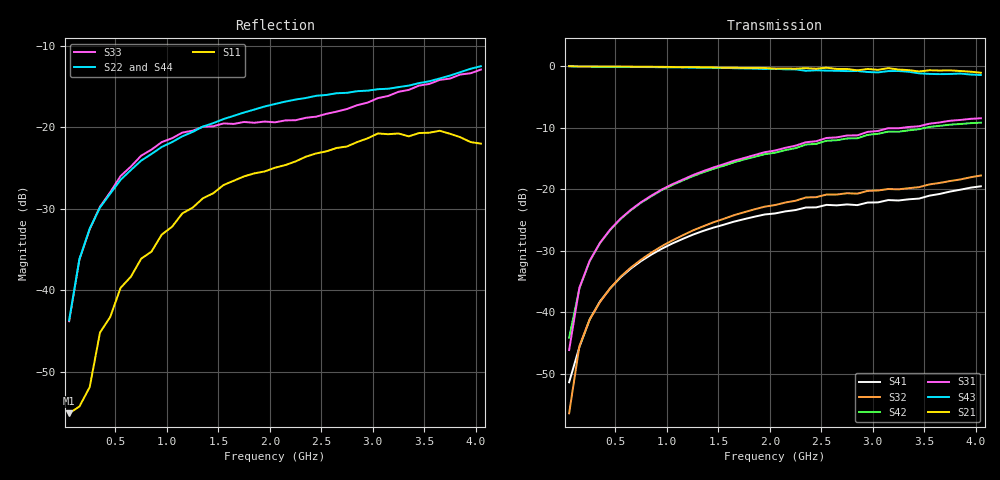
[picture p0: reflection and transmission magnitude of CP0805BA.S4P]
! Network Analyzer HP8720D.07.14 Serial No. US38111185
! 28 Apr 1999  02:06:29
! Frequency 	S11		S21		S31		S41		S12		S22		S23		S24		S13		S23		S33		S34		S14		S24		S34		S44
# HZ  S  DB R 50
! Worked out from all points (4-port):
!   41 points, 50 MHz to 4.05 GHz, reference 50 ohm
!   strongest paths, dB at 50 MHz, 1.05 GHz, 2.05 GHz, 3.05 GHz, 4.05 GHz:
!     S21: 0.0, -0.1, -0.4, -0.6, -1.0
!     S43: 0.0, -0.2, -0.4, -1.0, -1.4
!     S31: -46.1, -19.2, -13.7, -10.5, -8.4
!     S42: -44.1, -19.3, -14.0, -11.0, -9.1
!     S32: -56.4, -28.3, -22.5, -20.2, -17.7
!     S41: -51.3, -28.8, -23.9, -22.1, -19.5
!   lowest |S11| = -55.1 dB at 50 MHz (marker M1), VSWR 1.00, Z = 50.2 + j0.09 ohm
!   |S11| at or under -10 dB: start of sweep to end of sweep
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5e7  -55.07 30.6  0.00 -0.8  -46.45 85.9  -53.70 70.7
     0.04 -0.8  -43.67 61.7  -54.76 111.8  -44.55 83.9
     -46.11 96.2  -56.40 71.7  -43.78 50.0  0.00 -0.7
     -51.35 74.7  -44.09 87.6  0.03 -0.8  -43.67 61.7
1.5e8  -54.24 -71.2  0.01 -2.4  -35.96 87.7  -45.49 88.7
       -0.01 -2.5  -36.16 72.8  -45.68 89.2  -36.09 86.5
       -35.98 87.2  -45.47 88.7  -36.18 64.4  0.00 -2.9
       -45.61 90.3  -36.09 86.7  -0.01 -2.8  -36.16 72.8
2.5e8  -51.86 -91.4  -0.00 -4.2  -31.52 85.9  -41.13 86.1
       -0.01 -4.2  -32.43 72.8  -41.26 86.3  -31.62 85.4
       -31.60 85.5  -41.13 87.0  -32.49 60.8  -0.01 -4.7
       -41.12 86.8  -31.64 85.3  -0.02 -4.7  -32.43 72.8
5.5e8  -39.68 -108.5  -0.02 -9.1  -24.75 80.5  -34.28 81.2
       -0.03 -9.1  -26.43 70.8  -34.22 84.1  -24.81 80.1
       -24.73 80.6  -34.19 84.1  -25.96 48.9  -0.06 -10.3
       -34.29 81.2  -24.82 80.1  -0.07 -10.3  -26.43 70.8
9.5e8  -33.15 -135.1  -0.07 -15.8  -20.02 73.9  -29.61 74.4
       -0.07 -15.8  -22.40 63.4  -29.23 78.7  -20.13 73.1
       -20.01 73.7  -29.23 78.5  -21.80 31.9  -0.13 -17.6
       -29.64 74.1  -20.11 73.1  -0.13 -17.5  -22.40 63.4
3.05e9  -20.75 133.6  -0.52 -50.1  -10.45 37.1  -21.87 44.2
        -0.56 -49.6  -15.31 8.3  -20.22 42.4  -10.80 37.3
        -10.49 39.7  -20.17 45.1  -16.41 -54.3  -0.67 -55.4
        -22.10 46.2  -10.95 39.2  -0.97 -55.8  -15.31 8.3
4.05e9  -21.99 65.6  -0.89 -66.4  -8.20 21.2  -18.98 43.5
        -1.02 -66.9  -12.49 -48.6  -17.63 39.0  -8.77 21.8
        -8.43 24.2  -17.73 42.5  -12.91 -93.8  -0.96 -73.3
        -19.48 45.1  -9.14 24.1  -1.39 -74.7  -12.49 -48.6
